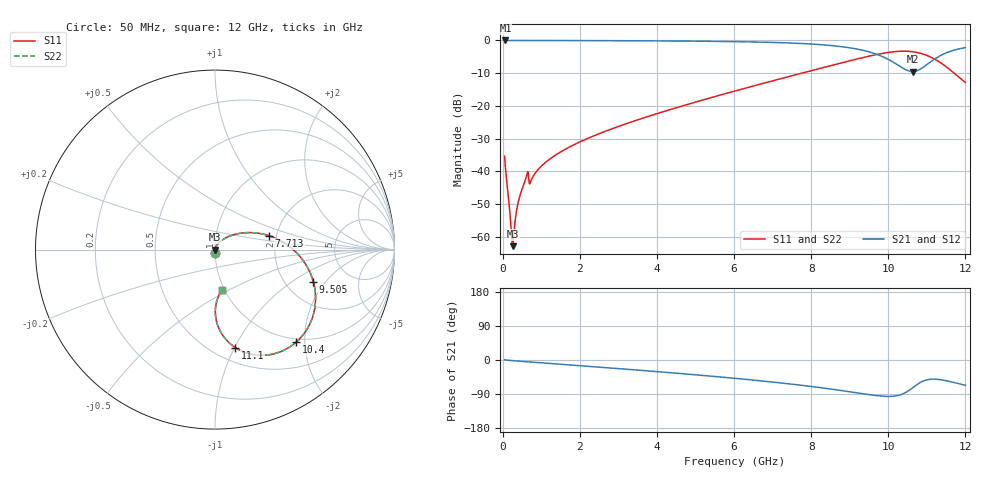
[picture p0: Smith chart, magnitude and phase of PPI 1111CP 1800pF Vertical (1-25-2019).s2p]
# GHz S MA R 50
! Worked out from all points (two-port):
!   1601 points, 50 MHz to 12 GHz, reference 50 ohm
!   highest |S21| = 0.00 dB at 72.41 MHz (marker M1); lowest = -9.5 dB at 10.63 GHz (marker M2)
!   |S21| within 3 dB of the highest: start of sweep to 9.341 GHz; 11.69 GHz to end of sweep
!   lowest |S11| = -62.9 dB at 259.1 MHz (marker M3), VSWR 1.00, Z = 50.1 - j6.53e-05 ohm
!   |S11| at or under -10 dB: start of sweep to 7.755 GHz; 11.71 GHz to end of sweep
!   |S22| runs from -62.9 to -3.3 dB; largest |S21 - S12| = 0
!   S11 on the Smith chart (normalised r, x): 50 MHz: 1.00, -0.03; 7.713 GHz: 1.83, +0.31; 9.505 GHz: 2.83, -1.51; 10.4 GHz: 0.94, -1.82; 11.1 GHz: 0.64, -1.01; 12 GHz: 0.97, -0.46
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0.05  0.01702 -88.1  0.9995 0.6  0.9995 0.6  0.01702 -88.1
0.07240625  0.01126 -87.7  0.9995 0.2  0.9995 0.2  0.01126 -87.7
0.2143125  0.001453 -64.5  0.9993 -1.4  0.9993 -1.4  0.001453 -64.5
0.259125  0.00072 -0.1  0.9993 -1.7  0.9993 -1.7  0.00072 -0.1
0.2964688  0.001232 49.1  0.9992 -2.0  0.9992 -2.0  0.001232 49.1
0.4159687  0.003628 71.9  0.999 -3.0  0.999 -3.0  0.003628 71.9
0.6101562  0.008133 72.5  0.9981 -4.5  0.9981 -4.5  0.008133 72.5
0.737125  0.007235 69.4  0.998 -5.3  0.998 -5.3  0.007235 69.4
1.177781  0.01473 72.8  0.9977 -8.7  0.9977 -8.7  0.01473 72.8
2.044156  0.02893 66.4  0.9953 -15.3  0.9953 -15.3  0.02893 66.4
4.038312  0.0774 50.0  0.9846 -30.9  0.9846 -30.9  0.0774 50.0
6.025  0.1691 32.7  0.9592 -48.3  0.9592 -48.3  0.1691 32.7
7.712937  0.3116 14.3  0.9003 -66.3  0.9003 -66.3  0.3116 14.3
8.019156  0.3473 10.2  0.8804 -70.1  0.8804 -70.1  0.3473 10.2
8.83325  0.4617 -3.1  0.7976 -81.3  0.7976 -81.3  0.4617 -3.1
9.505437  0.576 -18.0  0.6686 -91.4  0.6686 -91.4  0.576 -18.0
10.01331  0.6572 -33.6  0.509 -96.2  0.509 -96.2  0.6572 -33.6
10.40169  0.6857 -48.7  0.3709 -88.4  0.3709 -88.4  0.6857 -48.7
10.63322  0.6724 -58.7  0.3342 -73.2  0.3342 -73.2  0.6724 -58.7
11.09628  0.5579 -78.2  0.4708 -50.8  0.4708 -50.8  0.5579 -78.2
11.50706  0.3945 -89.0  0.6482 -54.8  0.6482 -54.8  0.3945 -89.0
12  0.2287 -80.4  0.7758 -66.7  0.7758 -66.7  0.2287 -80.4
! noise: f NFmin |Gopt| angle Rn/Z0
0.05  0.0004133  0.8786  0.3439  0.0007363
1.372  0.005742  0.7747  9.153  0.005176
2.701  0.01256  0.798  17.9  0.01257
4.031  0.02108  0.8226  26.42  0.02365
5.36  0.03131  0.8449  34.63  0.03911
6.682  0.04423  0.8673  42.44  0.0623
8.012  0.06448  0.8946  49.9  0.1097
9.341  0.1171  0.9345  56.97  0.3078
10.67  0.3817  0.9778  63.67  2.834
12  0.1502  0.9415  69.85  0.3857
